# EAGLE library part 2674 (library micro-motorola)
MICROCONTROLLER/MEMORY DEVICE
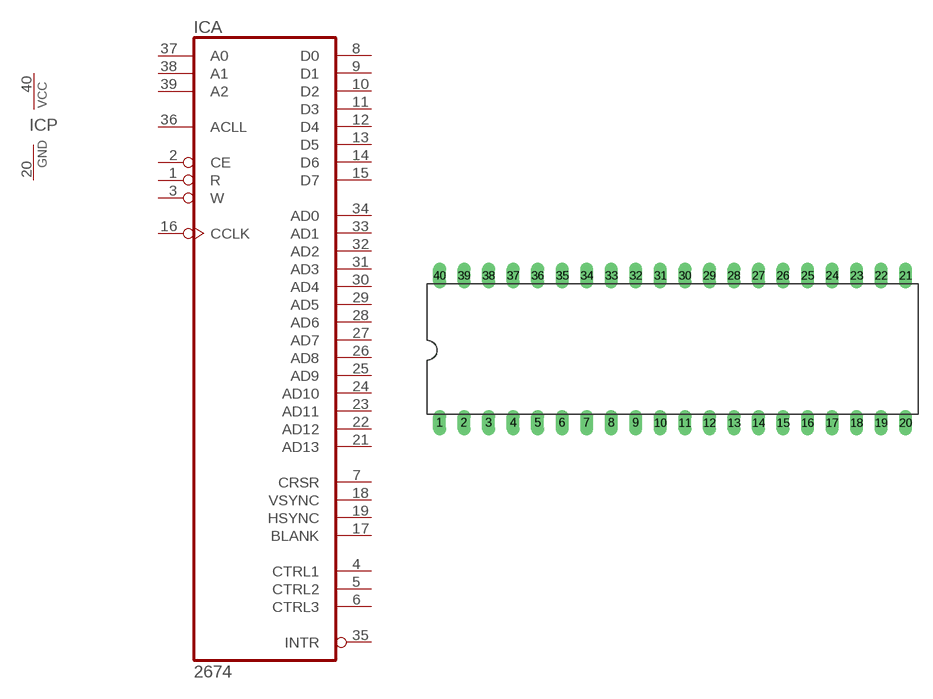
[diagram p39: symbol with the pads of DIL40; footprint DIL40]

Designator prefix IC; gates A=2674 P=PWRN

## 2674 (OC_FARNELL: unknown; OC_NEWARK: unknown)  [DIL40]
1  A:R  in
2  A:CE  in
3  A:W  in
4  A:CTRL1
5  A:CTRL2  out
6  A:CTRL3  out
7  A:CRSR  out
8  A:D0
9  A:D1
10  A:D2
11  A:D3
12  A:D4
13  A:D5
14  A:D6
15  A:D7
16  A:CCLK  in
17  A:BLANK  out
18  A:VSYNC  out
19  A:HSYNC  out
20  P:GND  pwr
21  A:AD13  out
22  A:AD12  out
23  A:AD11  out
24  A:AD10  out
25  A:AD9  out
26  A:AD8  out
27  A:AD7  out
28  A:AD6  out
29  A:AD5  out
30  A:AD4  out
31  A:AD3  out
32  A:AD2  out
33  A:AD1  out
34  A:AD0  out
35  A:INTR  out
36  A:ACLL  in
37  A:A0  in
38  A:A1  in
39  A:A2  in
40  P:VCC  pwr

## Footprint DIL40 (pad centres in mm)
Dual In Line Package
drill 0.813 long: 1 -24.13,-7.62; 2 -21.59,-7.62; 3 -19.05,-7.62; 4 -16.51,-7.62; 5 -13.97,-7.62; 6 -11.43,-7.62; 7 -8.89,-7.62; 8 -6.35,-7.62; 9 -3.81,-7.62; 10 -1.27,-7.62; 11 1.27,-7.62; 12 3.81,-7.62; 13 6.35,-7.62; 14 8.89,-7.62; 15 11.43,-7.62; 16 13.97,-7.62; 17 16.51,-7.62; 18 19.05,-7.62; 19 21.59,-7.62; 20 24.13,-7.62; 21 24.13,7.62; 22 21.59,7.62; 23 19.05,7.62; 24 16.51,7.62; 25 13.97,7.62; 26 11.43,7.62; 27 8.89,7.62; 28 6.35,7.62; 29 3.81,7.62; 30 1.27,7.62; 31 -1.27,7.62; 32 -3.81,7.62; 33 -6.35,7.62; 34 -8.89,7.62; 35 -11.43,7.62; 36 -13.97,7.62; 37 -16.51,7.62; 38 -19.05,7.62; 39 -21.59,7.62; 40 -24.13,7.62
